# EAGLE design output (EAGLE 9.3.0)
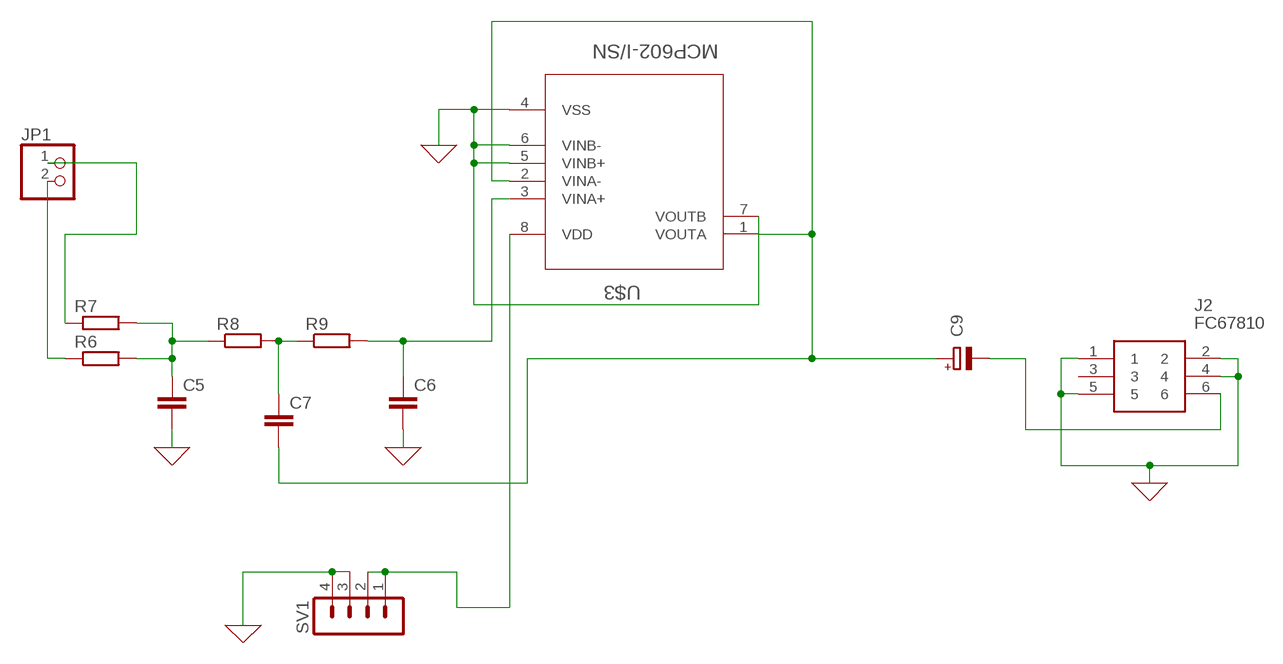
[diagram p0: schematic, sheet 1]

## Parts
C5  C-EUC0805  [C0805]
C6  C-EUC0805  [C0805]
C7  C-EUC0805  [C0805]
C9  CPOL-EUE2-5  [E2-5]
J2  FC67810  [FC67810]
JP1  PINHD-1X2  [1X02]
R6  R-EU_R0805  [R0805]
R7  R-EU_R0805  [R0805]
R8  R-EU_R0805  [R0805]
R9  R-EU_R0805  [R0805]
SV1  MA04-1  [MA04-1]
U$3  MCP602-I/SN  [SOIC127P600X175-8N]

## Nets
0: C5.2 C6.2 J2.1 J2.2 J2.4 J2.5 SV1.3 SV1.4 U$3.4(VSS) U$3.5(VINB+) U$3.6(VINB-) U$3.7(VOUTB) ; supply symbol labelled GND
N$1: C9.- J2.6
N$2: SV1.1 SV1.2 U$3.8(VDD)
N$12: C5.1 R6.2 R7.2 R8.1
N$14: JP1.1 R7.1
N$15: JP1.2 R6.1
N$16: C7.1 R8.2 R9.1
N$17: C6.1 R9.2 U$3.3(VINA+)
N$19: C7.2 C9.+ U$3.1(VOUTA) U$3.2(VINA-)
Unconnected: J2.3

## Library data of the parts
C5-C7 = rcl:C-EU: CAPACITOR, European symbol; SPICEPREFIX: C
C9 = rcl:CPOL-EU: POLARIZED CAPACITOR, European symbol; SPICEPREFIX: C
J2 = SamacSys_Parts:FC67810: S1K,Sealed jack sockets, stereo 1/4" Cliff Electronics 6.35mm PCB Mount Stereo Jack Socket, 5A Source: Datasheet; DESCRIPTION: S1K,Sealed jack sockets, stereo 1/4" Cliff Electronics 6.35mm PCB Mount Stereo Jack Socket, 5A; HEIGHT: mm; MANUFACTURER_NAME: CLIFF ELECTRONIC COMPONENTS; MANUFACTURER_PART_NUMBER: FC67810; MOUSER_PART_NUMBER: 8051646; MOUSER_PRICE-STOCK: http://uk.rs-online.com/web/p/products/8051646; RS_PART_NUMBER: 8051646; RS_PRICE-STOCK: http://uk.rs-online.com/web/p/products/8051646
JP1 = pinhead:PINHD-1X2: PIN HEADER
R6-R9 = rcl:R-EU_: RESISTOR, European symbol; SPICEPREFIX: R
SV1 = con-lstb:MA04-1: PIN HEADER; OC_FARNELL: unknown; OC_NEWARK: unknown
U$3 = Microchip_By_element14_Batch_1:MCP602-I/SN: CMOS Op Amp; MPN: MCP602-I/SN; OC_FARNELL: 9758666; OC_NEWARK: 12C1813;; PACKAGE: SOIC-8; SUPPLIER: Microchip

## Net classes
0 default: width 0.305 mm, drill 0.762 mm, clearance 0.508 mm

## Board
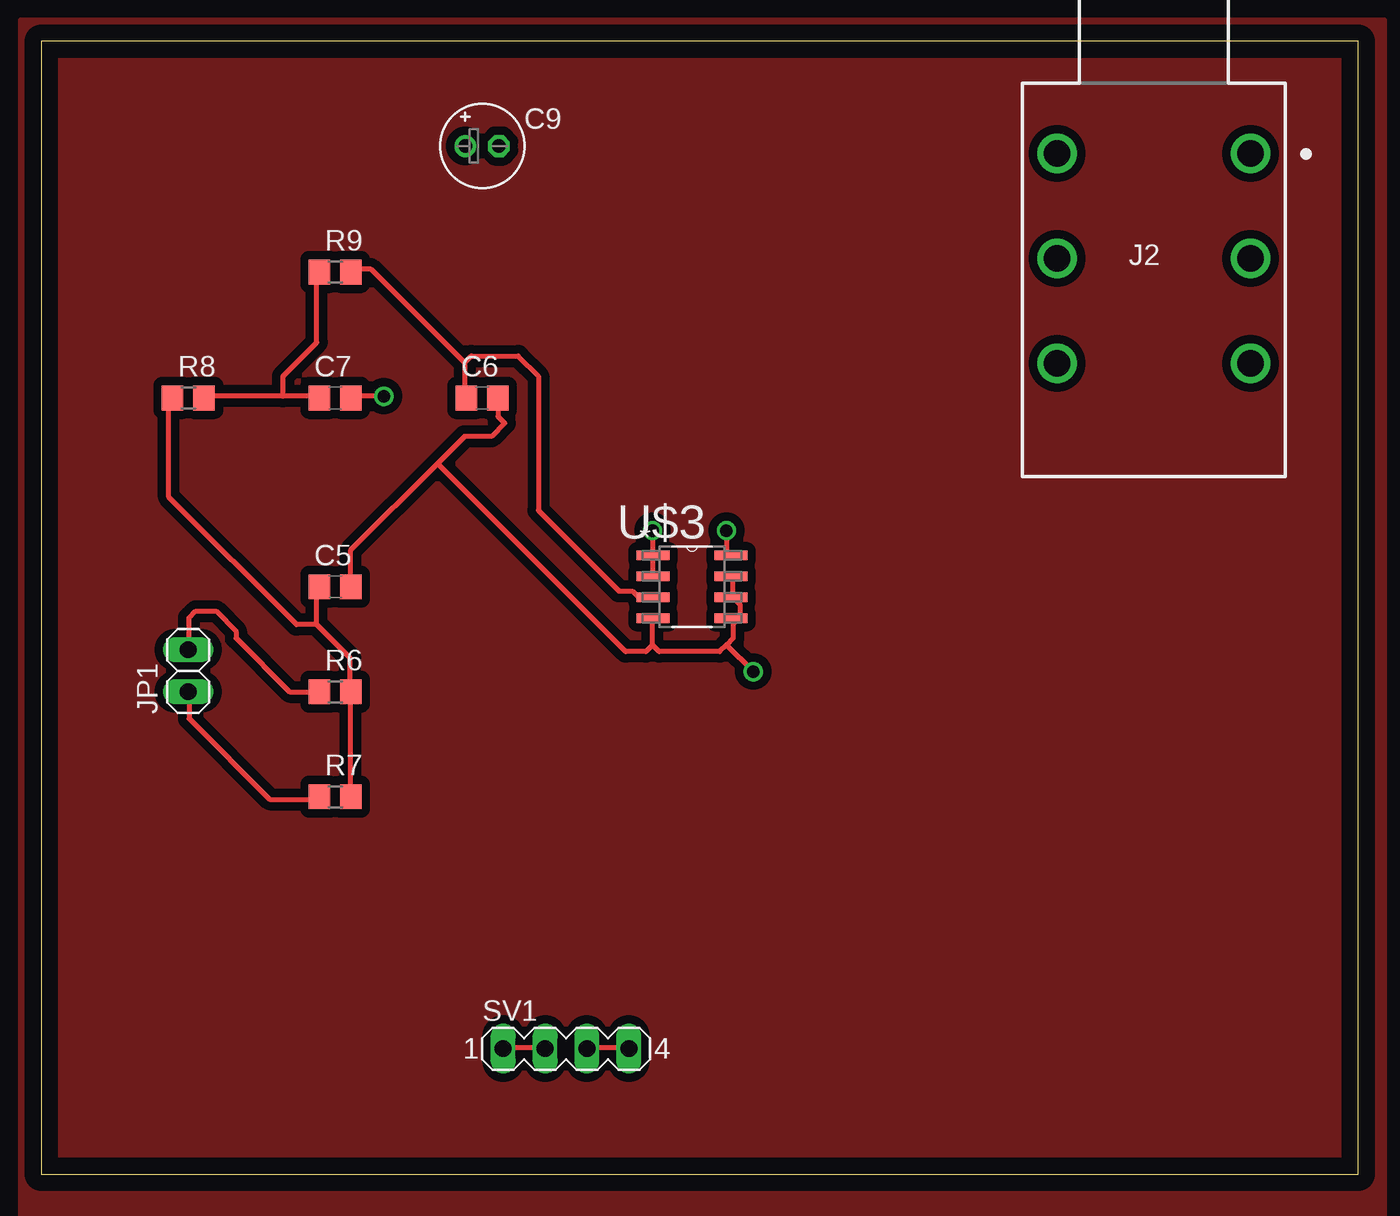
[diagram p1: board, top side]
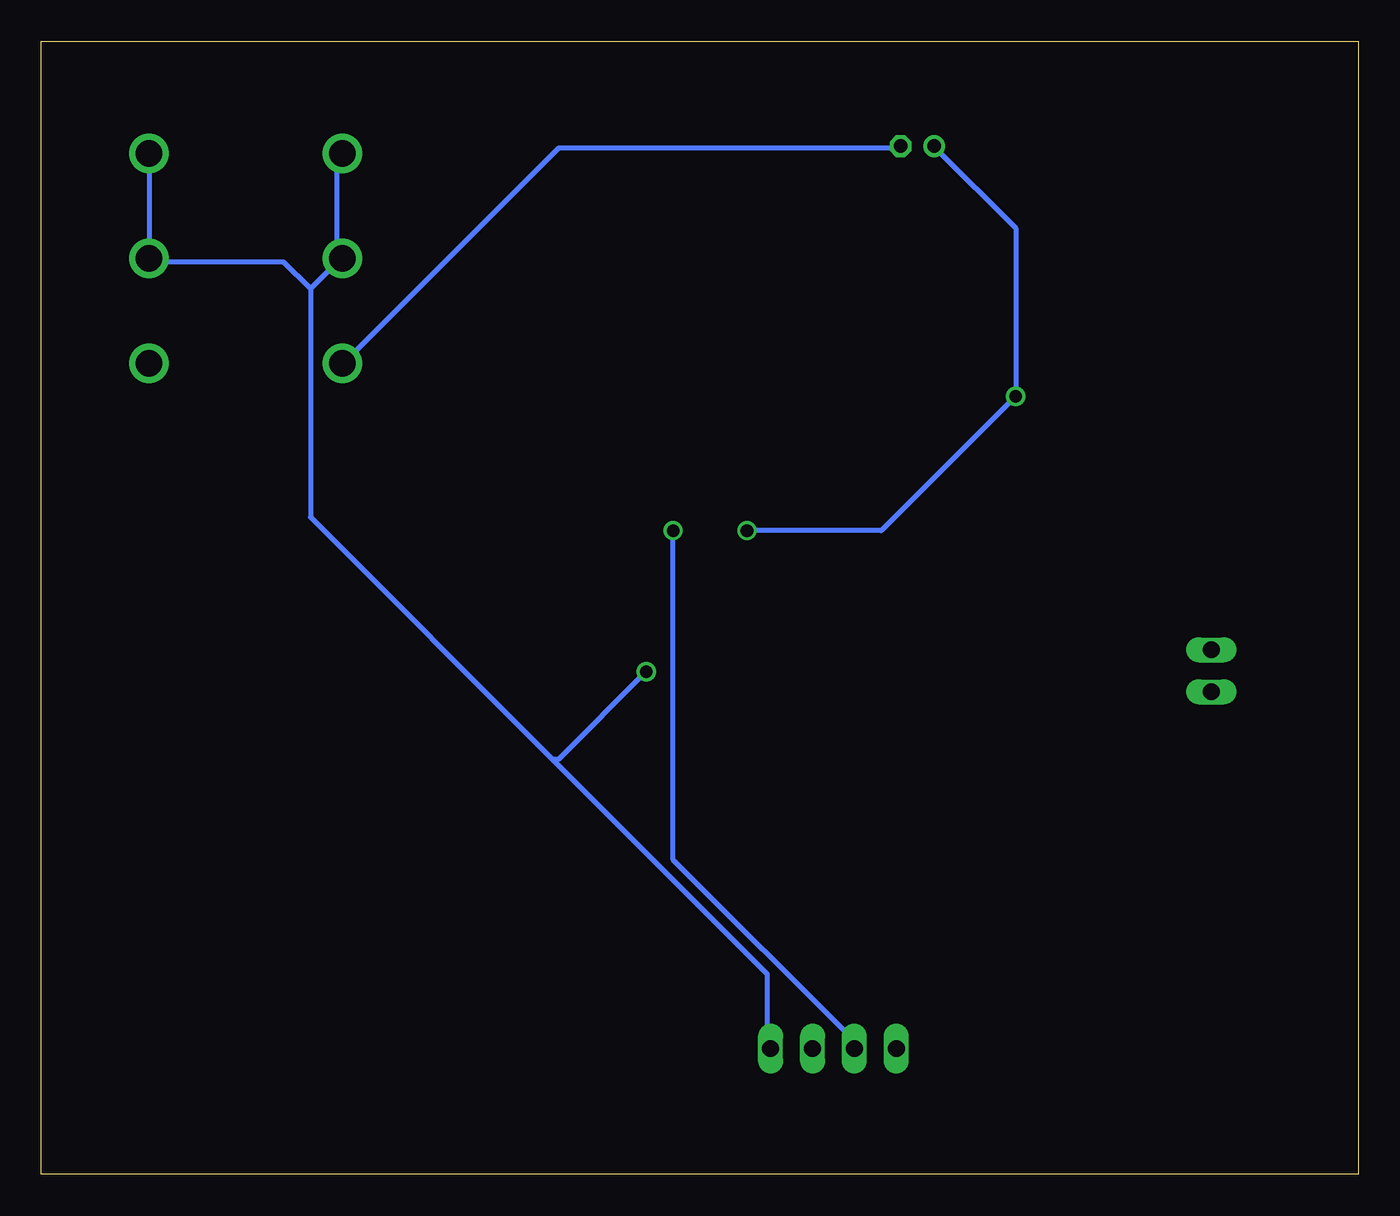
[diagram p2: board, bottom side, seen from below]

Size 79.68 x 68.57 mm. Coordinates in mm from the lower left corner, seen from the top.
Outline: 0,0 79.68,0 79.68,68.57 0,68.57 0,0
Copper layers (1*16): Top 0.035mm / dielectric 1.5mm / Bottom 0.035mm
Design rules "default": minimum track width 6mil, minimum drill 0.35mm, track to track 6mil, track to pad 6mil, pad to pad 6mil, via to via 6mil, smd to smd 6mil, copper to edge 40mil, drill to drill 6mil, minimum pad ring 10mil, minimum via ring 8mil, stop-mask expansion 4mil, vias tented up to drill 0mil, thermal gap 10mil

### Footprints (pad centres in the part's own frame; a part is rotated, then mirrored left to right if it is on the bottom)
C0805 = smd 1.3 x 1.5: 1 -0.95,0; 2 0.95,0
E2-5 = drill 0.813 pad 1.27: + -1.016,0 | drill 0.813 pad 1.27 octagon: - 1.016,0
FC67810 = drill 1.6 pad 2.4: 1 5.85,-4.25; 2 5.85,-10.6; 3 5.85,-16.95; 4 -5.85,-4.25; 5 -5.85,-10.6; 6 -5.85,-16.95
1X02 = drill 1.016 long: 1 -1.27,0; 2 1.27,0
R0805 = smd 1.3 x 1.5: 1 -0.95,0; 2 0.95,0
MA04-1 = drill 1.016 long: 1 -3.81,0; 2 -1.27,0; 3 1.27,0; 4 3.81,0
SOIC127P600X175-8N = smd 1.981 x 0.559: 1 -2.362,1.905; 2 -2.362,0.635; 3 -2.362,-0.635; 4 -2.362,-1.905; 5 2.362,-1.905; 6 2.362,-0.635; 7 2.362,0.635; 8 2.362,1.905

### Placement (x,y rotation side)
C5  17.78,35.56 0 top
C6  26.67,46.99 0 top
C7  17.78,46.99 0 top
C9  26.67,62.23 0 top
J2  67.31,66.04 0 top
JP1  8.89,30.48 90 top
R6  17.78,29.21 0 top
R7  17.78,22.86 0 top
R8  8.89,46.99 0 top
R9  17.78,54.61 0 top
SV1  31.75,7.62 0 top
U$3  39.37,35.56 0 top

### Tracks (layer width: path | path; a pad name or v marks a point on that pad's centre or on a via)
0  (via drill 0.76)
  Top 0.305: 23.98,43.03 25.6,44.65 27.23,44.65 28.04,45.47 27.63,45.87 27.63,46.28 28.04,46.69 27.63,47.09 C6.2 | 23.98,43.03 18.69,37.74 18.69,35.71 C5.2 | 36.98,32.05 36.98,33.68 U$3.4 | 36.98,32.05 37.39,31.65 41.05,31.65 41.45,32.05 | 41.45,32.05 41.86,32.46 41.86,33.27 42.27,33.68 | 42.27,33.68 42.27,34.49 41.86,34.9 | 42.27,33.68 41.86,33.68 U$3.5 | 41.86,34.9 41.86,36.12 U$3.7 | 41.86,34.9 U$3.6 | SV1.3 33.33,7.67 35.36,7.67 SV1.4 | v43.08,30.43 41.45,32.05 | 23.98,43.03 35.36,31.65 36.58,31.65 36.98,32.05
  Bottom 0.305: J2.1 73.15,61.72 73.15,55.63 J2.2 73.15,55.22 65.02,55.22 63.4,53.59 | 48.77,25.15 63.4,39.78 63.4,53.59 | 48.77,25.15 35.76,12.14 35.76,7.67 SV1.4 | 63.4,53.59 61.77,55.22 J2.5 61.77,55.63 61.77,61.72 J2.4 | v43.08,30.43 48.36,25.15 48.77,25.15
GND
  pour Top: -1.27,69.85 -1.27,-2.54 81.28,-2.54 81.28,69.85
N$1
  Bottom 0.305: C9.- 28.04,62.13 48.36,62.13 61.37,49.12 J2.6
N$2  (via drill 0.76)
  Top 0.305: v41.45,38.96 41.45,37.34 U$3.8 | SV1.1 28.04,7.67 30.48,7.67 SV1.2
  Bottom 0.305: v41.45,38.96 41.45,19.05 30.48,8.08 SV1.2
N$12
  Top 0.305: 18.69,29.21 18.69,23.11 R7.2 | 16.66,33.27 16.66,35.31 C5.1 | 16.66,33.27 18.69,31.24 18.69,29.21 | 18.69,29.21 R6.2 | 16.66,33.27 15.44,33.27 7.72,41 7.72,46.69 R8.1
N$14
  Top 0.305: R7.1 16.66,22.71 13.82,22.71 8.94,27.58 8.94,29.21 JP1.1
N$15
  Top 0.305: R6.1 15.04,29.21 11.79,32.46 11.79,32.87 10.57,34.09 9.35,34.09 8.94,33.68 8.94,32.46 9.35,32.05 8.94,31.65 JP1.2
N$16
  Top 0.305: 14.63,47.09 16.26,47.09 16.66,47.5 17.07,47.09 C7.1 | 14.63,47.09 10.16,47.09 R8.2 | 14.63,47.09 14.63,48.31 16.66,50.34 16.66,54.41 R9.1
N$17
  Top 0.305: 25.6,49.12 25.6,47.09 C6.1 | 25.6,49.12 19.91,54.81 19.1,54.81 R9.2 | 25.6,49.12 26.01,49.53 28.85,49.53 30.07,48.31 30.07,40.18 34.95,35.31 35.76,35.31 36.17,34.9 36.98,34.9 U$3.3
N$19  (via drill 0.76)
  Top 0.305: 36.98,37.34 36.98,36.12 U$3.2 | v20.73,47.09 19.1,47.09 C7.2 | v36.98,38.96 36.98,37.34 | 36.98,37.34 U$3.1
  Bottom 0.305: C9.+ 25.6,62.13 20.73,57.25 v20.73,47.09 28.85,38.96 v36.98,38.96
